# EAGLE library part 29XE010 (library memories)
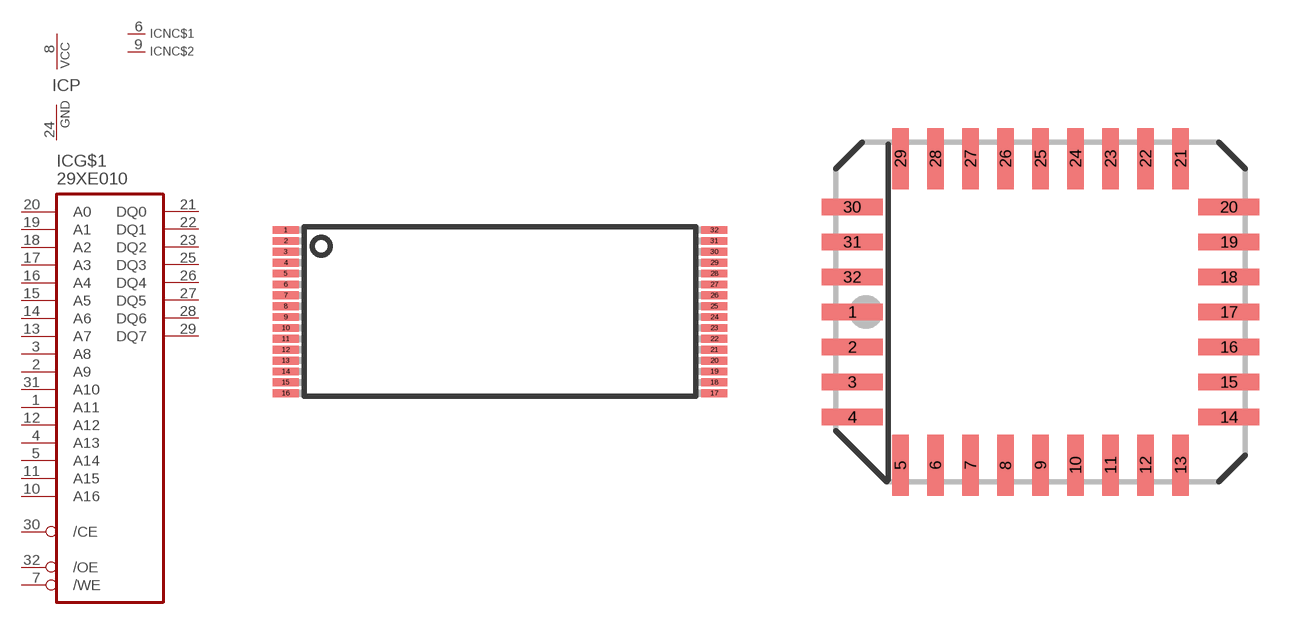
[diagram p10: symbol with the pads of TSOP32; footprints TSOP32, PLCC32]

Designator prefix IC; gates G$1=29EE010 P=PWRN NC$1=NC NC$2=NC

## 29XE010E  [TSOP32]
1  G$1:A11  in
2  G$1:A9  in
3  G$1:A8  in
4  G$1:A13  in
5  G$1:A14  in
6  NC$1:NC  nc
7  G$1:/WE  in
8  P:VCC  pwr
9  NC$2:NC  nc
10  G$1:A16  in
11  G$1:A15  in
12  G$1:A12  in
13  G$1:A7  in
14  G$1:A6  in
15  G$1:A5  in
16  G$1:A4  in
17  G$1:A3  in
18  G$1:A2  in
19  G$1:A1  in
20  G$1:A0  in
21  G$1:DQ0
22  G$1:DQ1
23  G$1:DQ2
24  P:GND  pwr
25  G$1:DQ3
26  G$1:DQ4
27  G$1:DQ5
28  G$1:DQ6
29  G$1:DQ7
30  G$1:/CE  in
31  G$1:A10  in
32  G$1:/OE  in

## 29XE010P  [PLCC32]
1  NC$1:NC  nc
2  G$1:A16  in
3  G$1:A15  in
4  G$1:A12  in
5  G$1:A7  in
6  G$1:A6  in
7  G$1:A5  in
8  G$1:A4  in
9  G$1:A3  in
10  G$1:A2  in
11  G$1:A1  in
12  G$1:A0  in
13  G$1:DQ0
14  G$1:DQ1
15  G$1:DQ2
16  P:GND  pwr
17  G$1:DQ3
18  G$1:DQ4
19  G$1:DQ5
20  G$1:DQ6
21  G$1:DQ7
22  G$1:/CE  in
23  G$1:A10  in
24  G$1:/OE  in
25  G$1:A11  in
26  G$1:A9  in
27  G$1:A8  in
28  G$1:A13  in
29  G$1:A14  in
30  NC$2:NC  nc
31  G$1:/WE  in
32  P:VCC  pwr

## 29XE010P-TH-SOCKET  [PLCC-S32]
Pads as for PLCC32

## 29XE010P-SMT-SOCKET  [PLCCSM32]
Pads as for PLCC32

## 29XE010N  [DIL32-6]
Pads as for PLCC32

## Footprint TSOP32 (pad centres in mm)
smd 1.2 x 0.36: 1 -9.85,3.75; 2 -9.85,3.25; 3 -9.85,2.75; 4 -9.85,2.25; 5 -9.85,1.75; 6 -9.85,1.25; 7 -9.85,0.75; 8 -9.85,0.25; 9 -9.85,-0.25; 10 -9.85,-0.75; 11 -9.85,-1.25; 12 -9.85,-1.75; 13 -9.85,-2.25; 14 -9.85,-2.75; 15 -9.85,-3.25; 16 -9.85,-3.75; 17 9.85,-3.75; 18 9.85,-3.25; 19 9.85,-2.75; 20 9.85,-2.25; 21 9.85,-1.75; 22 9.85,-1.25; 23 9.85,-0.75; 24 9.85,-0.25; 25 9.85,0.25; 26 9.85,0.75; 27 9.85,1.25; 28 9.85,1.75; 29 9.85,2.25; 30 9.85,2.75; 31 9.85,3.25; 32 9.85,3.75

## Footprint PLCC32 (pad centres in mm)
PLASTIC LEADED CHIP CARRIER rectangle, package type L
smd 2.2 x 0.6: 1 -6.83,0; 2 -6.83,-1.27; 3 -6.83,-2.54; 4 -6.83,-3.81; 14 6.83,-3.81; 15 6.83,-2.54; 16 6.83,-1.27; 17 6.83,0; 18 6.83,1.27; 19 6.83,2.54; 20 6.83,3.81; 30 -6.83,3.81; 31 -6.83,2.54; 32 -6.83,1.27
smd 0.6 x 2.2: 5 -5.08,-5.56; 6 -3.81,-5.56; 7 -2.54,-5.56; 8 -1.27,-5.56; 9 0,-5.56; 10 1.27,-5.56; 11 2.54,-5.56; 12 3.81,-5.56; 13 5.08,-5.56; 21 5.08,5.56; 22 3.81,5.56; 23 2.54,5.56; 24 1.27,5.56; 25 0,5.56; 26 -1.27,5.56; 27 -2.54,5.56; 28 -3.81,5.56; 29 -5.08,5.56

## Footprint PLCC-S32 (pad centres in mm)
Plastic Leaded Chip Carrier Socket
drill 0.813: 1 1.27,5.08
drill 0.813 octagon: 2 -1.27,7.62; 3 -1.27,5.08; 4 -3.81,7.62; 5 -6.35,5.08; 6 -3.81,5.08; 7 -6.35,2.54; 8 -3.81,2.54; 9 -6.35,0; 10 -3.81,0; 11 -6.35,-2.54; 12 -3.81,-2.54; 13 -6.35,-5.08; 14 -3.81,-7.62; 15 -3.81,-5.08; 16 -1.27,-7.62; 17 -1.27,-5.08; 18 1.27,-7.62; 19 1.27,-5.08; 20 3.81,-7.62; 21 6.35,-5.08; 22 3.81,-5.08; 23 6.35,-2.54; 24 3.81,-2.54; 25 6.35,0; 26 3.81,0; 27 6.35,2.54; 28 3.81,2.54; 29 6.35,5.08; 30 3.81,7.62; 31 3.81,5.08; 32 1.27,7.62

## Footprint PLCCSM32 (pad centres in mm)
smd 0.66 x 2.591: 1 0,7.62; 2 -1.27,7.62; 3 -2.54,7.62; 4 -3.81,7.62; 14 -3.81,-7.62; 15 -2.54,-7.62; 16 -1.27,-7.62; 17 0,-7.62; 18 1.27,-7.62; 19 2.54,-7.62; 20 3.81,-7.62; 30 3.81,7.62; 31 2.54,7.62; 32 1.27,7.62
smd 2.591 x 0.66: 5 -6.35,5.08; 6 -6.35,3.81; 7 -6.35,2.54; 8 -6.35,1.27; 9 -6.35,0; 10 -6.35,-1.27; 11 -6.35,-2.54; 12 -6.35,-3.81; 13 -6.35,-5.08; 21 6.35,-5.08; 22 6.35,-3.81; 23 6.35,-2.54; 24 6.35,-1.27; 25 6.35,0; 26 6.35,1.27; 27 6.35,2.54; 28 6.35,3.81; 29 6.35,5.08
